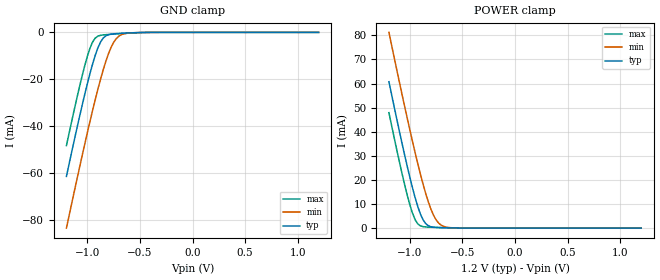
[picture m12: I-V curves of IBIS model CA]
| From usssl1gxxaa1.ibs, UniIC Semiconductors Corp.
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|   Model CA
[Model] CA
Model_type Input
Vinl =  0.500V
Vinh =  0.700V
C_comp   1.051pF   1.012pF   1.102pF
[Model Spec]
Vinh   0.700V   0.670V   0.750V
Vinl   0.500V   0.470V   0.550V
[Temperature Range]   25.000   0.125k   -40.000
[Voltage Range]   1.200V   1.140V   1.300V
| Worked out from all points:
|   GND clamp passes 1 mA (typ) near -0.80 V on its own axis
|   POWER clamp passes 1 mA (typ) near -0.83 V on its own axis
[GND_clamp]
|Voltage   I(typ)   I(min)   I(max)
-1.2V     -61.55mA   -83.64mA   -48.37mA
-1.05V    -31.07mA   -52.59mA   -18.49mA
-1V       -21.76mA   -42.69mA   -10.1mA
-950mV    -13.34mA   -33.17mA   -4.036mA
-900mV    -6.537mA   -24.18mA   -1.602mA
-850mV    -2.437mA   -16.01mA   -1.094mA
-775mV    -748.8uA   -6.382mA   -817.6uA
-750mV    -614.3uA   -4.205mA   -739.8uA
-700mV    -456uA     -1.582mA   -591.3uA
-625mV    -287.3uA   -381.3uA   -387.4uA
-475mV    -54.82uA   -45.05uA   -81.32uA
1.2V      0A         0A         0A
[POWER_clamp]
|Voltage   I(typ)   I(min)   I(max)
-1.2V     60.73mA    81.22mA    47.9mA
-1.125V   45.16mA    65.61mA    32.4mA
-1.05V    30.24mA    50.4mA     17.95mA
-1V       20.92mA    40.6mA     9.554mA
-950mV    12.52mA    31.18mA    3.432mA
-900mV    5.796mA    22.33mA    945.4uA
-850mV    1.867mA    14.37mA    492.9uA
-775mV    372.7uA    5.291mA    339.2uA
-750mV    278.4uA    3.357mA    302.5uA
-700mV    190.2uA    1.161mA    234.9uA
-525mV    46.75uA    52.32uA    57.81uA
1.2V      0A         0A         0A
